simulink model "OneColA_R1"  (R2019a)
settings: Solver=ode15s  StartTime=0.0  StopTime=tend  RelTol=1e-3
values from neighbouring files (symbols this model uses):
  Extract_J = zeros(83,1)'    [Simulate1Col.m]    (also in Simulate1Col_OL.m; Simulate1Col_R1.m; Simulate1Col_R2.m)
  Extract_xB = zeros(82,1)'    [Simulate1Col.m]    (also in Simulate1Col_OL.m; Simulate1Col_R1.m; Simulate1Col_R2.m)
  Extract_xD = zeros(82,1)'    [Simulate1Col.m]    (also in Simulate1Col_OL.m; Simulate1Col_R1.m; Simulate1Col_R2.m)
  F0 = 1    [colamod.m]    (also in ColumnA_simulation.m; Simulate1Col.m = F; Simulate1Col_OL.m = F; Simulate1Col_R1.m = F)
  F0step = 0.05    [Simulate1Col.m]    (also in Simulate1Col_OL.m = 1*F0*.1; Simulate1Col_R1.m; Simulate1Col_R2.m = 0.15)
  F0step2 = 0*(0.15-F0step)    (= 0)    [Simulate1Col.m]    (also in Simulate1Col_R1.m; Simulate1Col_R2.m = 0.1)
  F0step2_t = 30    [Simulate1Col.m]    (also in Simulate1Col_R1.m; Simulate1Col_R2.m = 80)
  F0step_t = 10    [Simulate1Col.m]    (also in Simulate1Col_OL.m; Simulate1Col_R1.m; Simulate1Col_R2.m)
  Kc_LTxD = tau_LTxD /(K_LTxD *(tauc_LTxD+theta_LTxD))    (= 23.0752764867)    [TuningCol.m]
  Kc_VxB = tau_VxB /(K_VxB *(tauc_VxB+theta_VxB))    (= 83.8414634146)    [TuningCol.m]
  KI_LTxD = Kc_LTxD/tauI_LTxD    [TuningCol.m]
  KI_VxB = Kc_VxB/tauI_VxB    [TuningCol.m]
  LmaxPI = Lmax-LT0    [Simulate1Col.m]    (also in Simulate1Col_R1.m; Simulate1Col_R2.m)
  LT0 = u_opt(1)    [Simulate1Col.m]    (also in Simulate1Col_OL.m; Simulate1Col_R1.m; Simulate1Col_R2.m)
  pV0 = pV    [Simulate1Col.m]    (also in Simulate1Col_OL.m; Simulate1Col_R1.m; Simulate1Col_R2.m)
  pVstep = 0.02    [Simulate1Col.m]    (also in Simulate1Col_OL.m = 0*(0.13-pV0); Simulate1Col_R1.m; Simulate1Col_R2.m = 0.06)
  pVstept = 50    [Simulate1Col.m]    (also in Simulate1Col_OL.m; Simulate1Col_R1.m; Simulate1Col_R2.m)
  qF = U(7)    [colamod.m]    (also in ColumnA_simulation.m; Simulate1Col.m = 1; Simulate1Col_OL.m = 1; Simulate1Col_R1.m = 1)
  VB0 = u_opt(2)    [Simulate1Col.m]    (also in Simulate1Col_OL.m; Simulate1Col_R1.m; Simulate1Col_R2.m)
  VmaxPI = Vmax-VB0    [Simulate1Col.m]    (also in Simulate1Col_R1.m; Simulate1Col_R2.m)
  x0 = 0.5*ones(1,82)'    [col_obj.m]    (also in Simulate1Col.m = x; Simulate1Col_OL.m = x; Simulate1Col_R1.m = x; Simulate1Col_R2.m = x)
  xBsp = 0.95    [Simulate1Col.m]    (also in Simulate1Col_OL.m; Simulate1Col_R1.m; Simulate1Col_R2.m)
  xDmin = 0.95    [Simulate1Col.m]    (also in Simulate1Col_OL.m; Simulate1Col_R1.m; Simulate1Col_R2.m)
  zF = U(6)    [colamod.m]    (also in ColumnA_simulation.m; Simulate1Col.m = 0.5; Simulate1Col_OL.m = 0.5; Simulate1Col_R1.m = 0.5)
undefined symbols (not defined in the file or in its folder): Calc_xDsp, ColumnA_simulation, extract
libraries: simulink x2

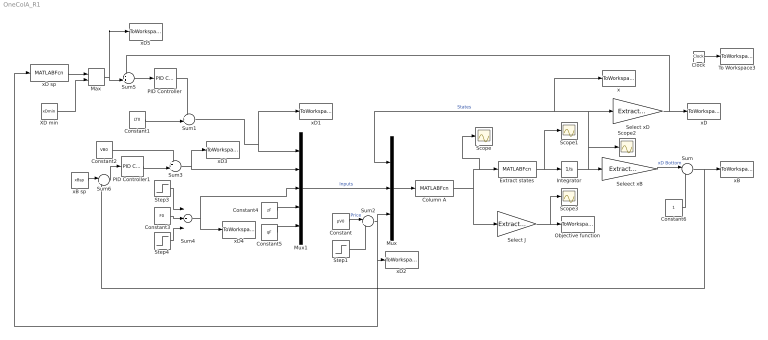
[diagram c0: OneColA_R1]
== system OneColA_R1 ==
  Clock : Clock
  Column A : MATLABFcn  MATLABFcn=ColumnA_simulation(u)  OutputDimensions=83
  Constant : Constant  Value=pV0
  Constant1 : Constant  Value=LT0
  Constant2 : Constant  Value=VB0
  Constant3 : Constant  Value=F0
  Constant4 : Constant  Value=zF
  Constant5 : Constant  Value=qF
  Constant6 : Constant
  Extract states : MATLABFcn  MATLABFcn=extract(u)  OutputDimensions=82
  Integrator : Integrator  InitialCondition=x0
  Max : MinMax  Function=max  Inputs=2
  Mux : Mux  Inputs=3
  Mux1 : Mux  Inputs=5
  Objective function : ToWorkspace  VariableName=Jactual  SampleTime=-1
  PID Controller : simulink/Continuous/PID Controller  Controller=PI  Form=Parallel  TimeDomain=Continuous-time  SampleTime=-1  IntegratorMethod=Forward Euler  FilterMethod=Forward Euler  ControllerParametersSource=internal  P=Kc_LTxD  I=KI_LTxD  D=0  UseFilter=on  N=100  TunerSelectOption=Transfer Function Based (PID Tuner App)  InitialConditionSource=internal  InitialConditionForIntegrator=0  InitialConditionForFilter=0  DifferentiatorICPrevScaledInput=0  ExternalReset=none  TrackingMode=off  Kt=1  LimitOutput=on  UpperSaturationLimit=LmaxPI  LowerSaturationLimit=-LT0  LinearizeAsGain=on  AntiWindupMode=none  Kb=1  POutMin=[]  POutMax=[]  IOutMin=[]  IOutMax=[]  DOutMin=[]  DOutMax=[]  NOutMin=[]  NOutMax=[]  SumOutMin=[]  SumOutMax=[]  SaturationOutMin=[]  SaturationOutMax=[]  PParamMin=[]  PParamMax=[]  IParamMin=[]  IParamMax=[]  DParamMin=[]  DParamMax=[]  NParamMin=[]  NParamMax=[]  KbParamMin=[]  KbParamMax=[]  KtParamMin=[]  KtParamMax=[]  KbOutMin=[]  KbOutMax=[]  KtOutMin=[]  KtOutMax=[]  IntegratorOutMin=[]  IntegratorOutMax=[]  FilterOutMin=[]  FilterOutMax=[]  SumI1OutMin=[]  SumI1OutMax=[]  SumI2OutMin=[]  SumI2OutMax=[]  SumI3OutMin=[]  SumI3OutMax=[]  SumI4OutMin=[]  SumI4OutMax=[]  SumDOutMin=[]  SumDOutMax=[]  DifferentiatorOutMin=[]  DifferentiatorOutMax=[]  FilterDiffOutCoefMin=[]  FilterDiffOutCoefMax=[]  ReciprocalOutMin=[]  ReciprocalOutMax=[]  SumDenOutMin=[]  SumDenOutMax=[]  SumNumOutMin=[]  SumNumOutMax=[]  DivideOutMin=[]  DivideOutMax=[]  IntegratorContinuousStateAttributes=''  IntegratorStateMustResolveToSignalObject=off  IntegratorRTWStateStorageClass=Auto  FilterContinuousStateAttributes=''  FilterStateMustResolveToSignalObject=off  FilterRTWStateStorageClass=Auto  ParallelPVariant=InternalParameters  IdealPVariant=Disabled  IVariant=InternalParameters  DVariant=Disabled  IntegratorVariant=Continuous  SatVariant=Enabled  AWVariant=Passthrough  PCopyVariant=Disabled  TRVariant=Disabled  FdbkBlocksVariant=Forward  IdealPFdbkVariant=Disabled  SatFdbkVariant=Disabled  DerivativeFilterVariant=Disabled  NVariant=Disabled  NCopyVariant=Disabled_SignalSpec  FilterICVariant=Disabled  IntegratorICVariant=InternalICs  ExternalResetVariant=Disabled  TRSumVariant=Passthrough  SumFdbkVariant=Disabled  SumVariant=Sum_PI
  PID Controller1 : simulink/Continuous/PID Controller  Controller=PI  Form=Parallel  TimeDomain=Continuous-time  SampleTime=-1  IntegratorMethod=Forward Euler  FilterMethod=Forward Euler  ControllerParametersSource=internal  P=Kc_VxB  I=KI_VxB  D=0  UseFilter=on  N=100  TunerSelectOption=Transfer Function Based (PID Tuner App)  InitialConditionSource=internal  InitialConditionForIntegrator=0  InitialConditionForFilter=0  DifferentiatorICPrevScaledInput=0  ExternalReset=none  TrackingMode=off  Kt=1  LimitOutput=on  UpperSaturationLimit=VmaxPI  LowerSaturationLimit=-VB0  LinearizeAsGain=on  AntiWindupMode=none  Kb=1  POutMin=[]  POutMax=[]  IOutMin=[]  IOutMax=[]  DOutMin=[]  DOutMax=[]  NOutMin=[]  NOutMax=[]  SumOutMin=[]  SumOutMax=[]  SaturationOutMin=[]  SaturationOutMax=[]  PParamMin=[]  PParamMax=[]  IParamMin=[]  IParamMax=[]  DParamMin=[]  DParamMax=[]  NParamMin=[]  NParamMax=[]  KbParamMin=[]  KbParamMax=[]  KtParamMin=[]  KtParamMax=[]  KbOutMin=[]  KbOutMax=[]  KtOutMin=[]  KtOutMax=[]  IntegratorOutMin=[]  IntegratorOutMax=[]  FilterOutMin=[]  FilterOutMax=[]  SumI1OutMin=[]  SumI1OutMax=[]  SumI2OutMin=[]  SumI2OutMax=[]  SumI3OutMin=[]  SumI3OutMax=[]  SumI4OutMin=[]  SumI4OutMax=[]  SumDOutMin=[]  SumDOutMax=[]  DifferentiatorOutMin=[]  DifferentiatorOutMax=[]  FilterDiffOutCoefMin=[]  FilterDiffOutCoefMax=[]  ReciprocalOutMin=[]  ReciprocalOutMax=[]  SumDenOutMin=[]  SumDenOutMax=[]  SumNumOutMin=[]  SumNumOutMax=[]  DivideOutMin=[]  DivideOutMax=[]  IntegratorContinuousStateAttributes=''  IntegratorStateMustResolveToSignalObject=off  IntegratorRTWStateStorageClass=Auto  FilterContinuousStateAttributes=''  FilterStateMustResolveToSignalObject=off  FilterRTWStateStorageClass=Auto  ParallelPVariant=InternalParameters  IdealPVariant=Disabled  IVariant=InternalParameters  DVariant=Disabled  IntegratorVariant=Continuous  SatVariant=Enabled  AWVariant=Passthrough  PCopyVariant=Disabled  TRVariant=Disabled  FdbkBlocksVariant=Forward  IdealPFdbkVariant=Disabled  SatFdbkVariant=Disabled  DerivativeFilterVariant=Disabled  NVariant=Disabled  NCopyVariant=Disabled_SignalSpec  FilterICVariant=Disabled  IntegratorICVariant=InternalICs  ExternalResetVariant=Disabled  TRSumVariant=Passthrough  SumFdbkVariant=Disabled  SumVariant=Sum_PI
  Scope{,1..3} (4 alike) : Scope
  Select J : Gain  Gain=Extract_J  Multiplication=Matrix(K*u)
  Select xD : Gain  Gain=Extract_xD  Multiplication=Matrix(K*u)
  Seleect xB : Gain  Gain=Extract_xB  Multiplication=Matrix(K*u)
  Step1 : Step  Time=pVstept  After=pVstep  SampleTime=0
  Step3 : Step  Time=F0step_t  After=F0step  SampleTime=0
  Step4 : Step  Time=F0step2_t  After=F0step2  SampleTime=0
  Sum : Sum  Inputs=|-+
  Sum1 : Sum  Inputs=++|
  Sum2 : Sum  Inputs=|++
  Sum3 : Sum  Inputs=++|
  Sum4 : Sum  Inputs=+++
  Sum5 : Sum  Inputs=-+|
  Sum6 : Sum  Inputs=|+-
  To Workspace3 : ToWorkspace  VariableName=time  SampleTime=-1
  XD min : Constant  Value=xDmin
  x : ToWorkspace  VariableName=States  SampleTime=-1
  xB : ToWorkspace  VariableName=xB  SampleTime=-1
  xB sp : Constant  Value=xBsp
  xD : ToWorkspace  VariableName=xD  SampleTime=-1
  xD sp : MATLABFcn  MATLABFcn=Calc_xDsp(u)  OutputDimensions=1
  xD1 : ToWorkspace  VariableName=LT  SampleTime=-1
  xD2 : ToWorkspace  VariableName=pV  SampleTime=-1
  xD3 : ToWorkspace  VariableName=VB  SampleTime=-1
  xD4 : ToWorkspace  VariableName=Fin  SampleTime=-1
  xD5 : ToWorkspace  VariableName=xDsp  SampleTime=-1
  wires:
  Mux/1 -> Column A/1
  Mux1/1 -> Mux/2  "Inputs"
  Constant4/1 -> Mux1/4
  Constant5/1 -> Mux1/5
  Column A/1 -> Select J/1, Extract states/1, Scope/1
  Extract states/1 -> Scope1/1, Integrator/1
  Integrator/1 -> Seleect xB/1, Select xD/1, x/1, Mux/1, Scope2/1  "States"
  Select xD/1 -> Sum5/1, xD/1
  Select J/1 -> Scope3/1, Objective function/1
  Clock/1 -> To Workspace3/1
  Seleect xB/1 -> Sum/1  "xD Bottom"
  Sum/1 -> xB/1, Sum6/2
  Constant6/1 -> Sum/2
  Sum1/1 -> xD1/1, Mux1/1
  Sum2/1 -> xD2/1, xD sp/1, Mux/3
  Constant/1 -> Sum2/1  "Price"
  Sum3/1 -> Mux1/2, xD3/1
  Constant3/1 -> Sum4/2
  Sum4/1 -> xD4/1, Mux1/3
  Step3/1 -> Sum4/1
  Step1/1 -> Sum2/2
  PID Controller/1 -> Sum1/1
  Sum5/1 -> PID Controller/1
  Step4/1 -> Sum4/3
  Constant2/1 -> Sum3/1
  Constant1/1 -> Sum1/2
  PID Controller1/1 -> Sum3/2
  Sum6/1 -> PID Controller1/1
  xB sp/1 -> Sum6/1
  Max/1 -> xD5/1, Sum5/2
  xD sp/1 -> Max/1
  XD min/1 -> Max/2
